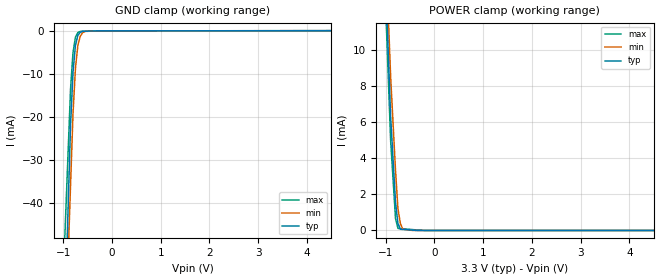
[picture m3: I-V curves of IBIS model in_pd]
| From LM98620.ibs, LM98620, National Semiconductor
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[Model] in_pd
Model_type Input
Vinl = 800.000mV
Vinh = 2.00000V
C_comp 876.000fF 822.000fF 926.000fF
| variable typ   min   max
[Voltage Range] 3.30000V 3.00000V 3.60000V
[POWER Clamp Reference] 3.30000V 3.00000V 3.60000V
[GND Clamp Reference] 0.00000V 0.00000V 0.00000V
[Temperature Range]   25   70   0
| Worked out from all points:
|   GND clamp passes 1 mA (typ) near -0.70 V on its own axis
|   POWER clamp passes 1 mA (typ) near -0.78 V on its own axis
[GND Clamp]
-3.3V     -959.2mA   -846.2mA   -729.1mA
-850mV    -21.73mA   -35.73mA   -13.38mA
-800mV    -9.601mA   -19.19mA   -5.032mA
-750mV    -3.361mA   -8.684mA   -1.466mA
-700mV    -1.009mA   -3.324mA   -393.9uA
-650mV    -329.3uA   -1.233mA   -122.4uA
-600mV    -98.69uA   -395.3uA   -105.1uA
-550mV    -83.11uA   -129.9uA   -87.66uA
-325mV    -13uA      -28.39uA   -9.393uA
-300mV    -5.208uA   -17.11uA   -9.128uA
-275mV    -4.976uA   -5.826uA   -8.863uA
6.6V      58.67uA    53.89uA    63.98uA
[POWER Clamp]
-3.3V     206.8mA    184.9mA    178.7mA
-1.05V    17.14mA    18.98mA    15.83mA
-900mV    6.302mA    8.515mA    4.97mA
-800mV    1.546mA    3.313mA    665.7uA
-750mV    392.8uA    1.204mA    114.3uA
-700mV    68.37uA    372.7uA    103.4uA
-650mV    58.6uA     78.02uA    92.55uA
-450mV    19.53uA    0A         49uA
-175mV    0A         0A         0A
6.6V      0A         0A         0A
